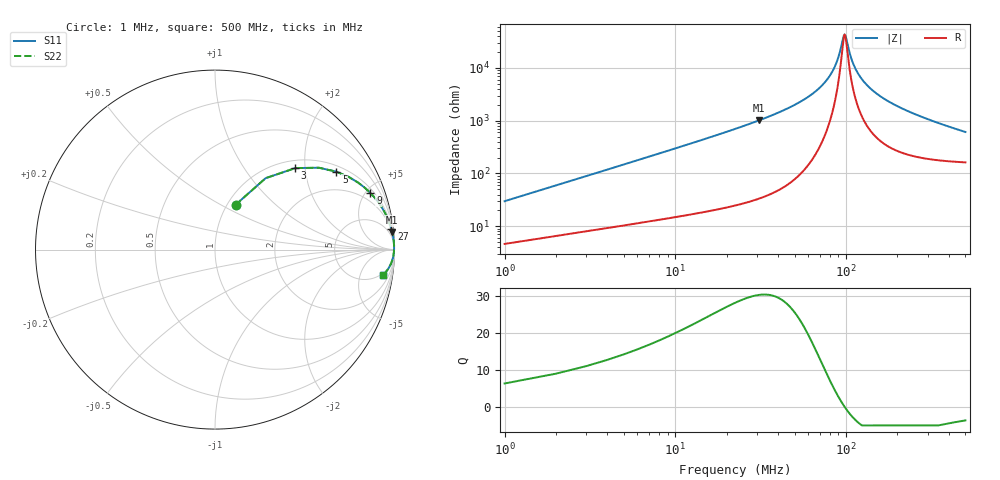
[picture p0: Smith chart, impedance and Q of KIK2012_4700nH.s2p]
!version-2
!date-01.2022
!Series
# MHz S RI R 50
!Freq ReS11 ImS11 ReS21 ImS21 ReS12 ImS12 ReS22 ImS22
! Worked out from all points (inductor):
!   500 points, 1 MHz to 500 MHz, reference 50 ohm
!   read as one part in series: L = 4.7 uH near 3 MHz
!   highest Q = 30.3 at 31 MHz (marker M1), where L = 5.22 uH
!   self-resonance near 98 MHz
!   S11 on the Smith chart (normalised r, x): 1 MHz: 1.09, +0.59; 3 MHz: 1.16, +1.77; 5 MHz: 1.21, +2.96; 9 MHz: 1.28, +5.36; 27 MHz: 2, +17; 500 MHz: 4, -12
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1  0.1148 0.2498  0.8852 -0.2498  0.8852 -0.2498  0.1148 0.2498
3  0.4469 0.454  0.5531 -0.454  0.5531 -0.454  0.4469 0.454
5  0.6763 0.4342  0.3237 -0.4342  0.3237 -0.4342  0.6763 0.4342
9  0.8656 0.3159  0.1344 -0.3159  0.1344 -0.3159  0.8656 0.3159
17  0.9574 0.1833  0.0426 -0.1833  0.0426 -0.1833  0.9574 0.1833
27  0.983 0.1134  0.017 -0.1134  0.017 -0.1134  0.983 0.1134
31  0.9873 0.0967  0.0127 -0.0967  0.0127 -0.0967  0.9873 0.0967
68  0.9975 0.0258  0.00246 -0.0258  0.00246 -0.0258  0.9975 0.0258
85  0.9979 0.00994  0.00211 -0.00994  0.00211 -0.00994  0.9979 0.00994
90  0.9979 0.00599  0.00215 -0.00599  0.00215 -0.00599  0.9979 0.00599
96  0.9977 0.00157  0.00227 -0.00157  0.00227 -0.00157  0.9977 0.00157
98  0.9977 0.000154  0.00232 -0.000154  0.00232 -0.000154  0.9977 0.000154
100  0.9976 -0.00123  0.00238 0.00123  0.00238 0.00123  0.9976 -0.00123
106  0.9974 -0.00522  0.00258 0.00522  0.00258 0.00522  0.9974 -0.00522
110  0.9973 -0.00775  0.00275 0.00775  0.00275 0.00775  0.9973 -0.00775
121  0.9967 -0.0143  0.0033 0.0143  0.0033 0.0143  0.9967 -0.0143
140  0.9955 -0.0246  0.00453 0.0246  0.00453 0.0246  0.9955 -0.0246
168  0.9931 -0.038  0.00687 0.038  0.00687 0.038  0.9931 -0.038
251  0.9833 -0.0713  0.0167 0.0713  0.0167 0.0713  0.9833 -0.0713
334  0.9702 -0.0987  0.0298 0.0987  0.0298 0.0987  0.9702 -0.0987
417  0.9544 -0.1221  0.0456 0.1221  0.0456 0.1221  0.9544 -0.1221
500  0.937 -0.1416  0.063 0.1416  0.063 0.1416  0.937 -0.1416
